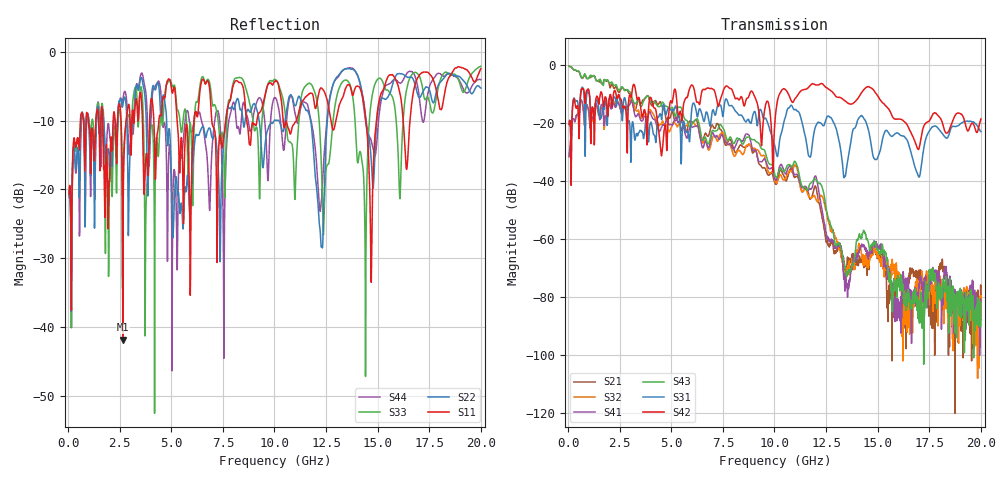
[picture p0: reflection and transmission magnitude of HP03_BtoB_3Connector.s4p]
# MHz S MA R 50.00
! FREQ  S11  S12  S13  S14
!  S21  S22  S23  S24
!  S31  S32  S33  S34
!  S41  S42  S43  S44
!  MAG  ANG  MAG  ANG  MAG  ANG  MAG  ANG
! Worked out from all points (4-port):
!   1996 points, 50 MHz to 20 GHz, reference 50 ohm
!   strongest paths, dB at 50 MHz, 5.04 GHz, 10.03 GHz, 15.02 GHz, 20 GHz:
!     S42: -20.5, -13.1, -18.8, -10.9, -18.7
!     S31: -20.5, -15.4, -28.4, -31.5, -23.0
!     S43: -0.5, -14.6, -38.3, -63.4, -81.8
!     S41: -31.6, -20.8, -39.5, -63.2, -87.7
!     S32: -31.6, -20.9, -40.0, -64.7, -86.7
!     S21: -0.5, -15.9, -40.8, -66.0, -83.1
!   lowest |S11| = -41.8 dB at 2.65 GHz (marker M1), VSWR 1.02, Z = 50.1 + j0.804 ohm
!   |S11| at or under -10 dB: 5.283 GHz to 6.097 GHz (814.6 MHz wide, 14.3 % of centre); 6.963 GHz to 7.643 GHz (680.5 MHz wide, 9.32 % of centre); 10.42 GHz to 11.06 GHz (639.6 MHz wide, 5.96 % of centre)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
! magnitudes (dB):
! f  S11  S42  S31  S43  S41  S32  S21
! 50 MHz  -20.6  -20.5  -20.5  -0.5  -31.6  -31.6  -0.5
! 2.65 GHz  -41.8  -14.8  -16.9  -7.8  -15.7  -15.5  -7.9
! 9.93 GHz  -4.7  -36.8  -26.7  -35.2  -36.7  -37.1  -38.4
! 12.27 GHz  -5.3  -6.4  -20.2  -41.4  -48.9  -45.3  -51.1
! 13.55 GHz  -4.8  -13.2  -32.9  -72.0  -77.1  -70.4  -67.4
! 14.4 GHz  -9.2  -8.1  -19.2  -58.2  -62.8  -68.6  -69.2
! 20 GHz  -2.4  -18.7  -23.0  -81.8  -87.7  -86.7  -83.1
